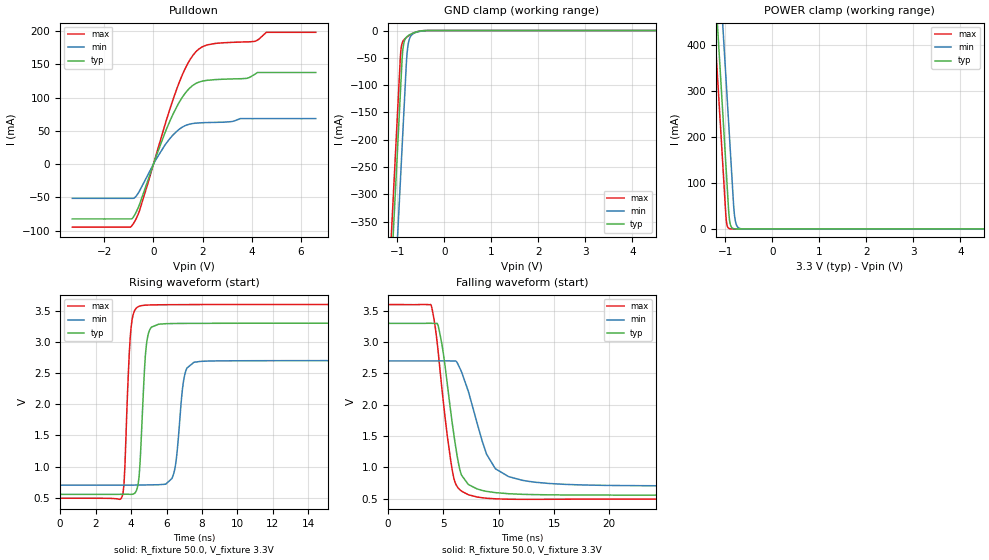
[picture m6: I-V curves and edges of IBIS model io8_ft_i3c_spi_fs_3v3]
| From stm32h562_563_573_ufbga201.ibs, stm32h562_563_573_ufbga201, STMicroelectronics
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[Model]   io8_ft_i3c_spi_fs_3v3
Model_type I/O_open_drain
Polarity   Non-Inverting
Enable   Active-Low
| CAP_THRESHOLD on pad IOFT is "UDTCAPC" :
| Rising=20.0% of vddiom   Falling=80.0% of vddiom
| C_comp min and max val. don't necessarily correlate with the min and max pvt
| but are the smallest and greatest pad capacitance found.
| var   typ   min   max
C_comp   3.95818pF  3.95027pF  4.00766pF
|C_comp_pulldown   3.95818pF  3.95027pF  4.00766pF
Vinl = 1.35V
Vinh = 1.8V
Vmeas = 1.65V   | Reference voltage for timing measurements
Cref  = 50.0pF   | Timing specification test load capacitance value
Rref  = 1.0MOhm   | Timing specification test load resistance value
Vref  = 1.815V   | Timing specification test load voltage
[Model Spec]
| TIME_THRESHOLD on pin ZII2CV11 is "CMOS" :
| Rising=40.0% of vdd   Falling=60.0% of vdd
Vinl 1.29880V 1.07480V 1.40680V
Vinh 1.77520V 1.49320V 1.89720V
| variable   typ   min   max
[Temperature Range] 25.0 125.0 -40.0
| variable   typ   min   max
[Voltage Range] 3.3V 2.7V 3.6V
| variable   typ   min   max
[POWER Clamp Reference] 3.3V 2.7V 3.6V
| variable   typ   min   max
[GND Clamp Reference] 0V 0V 0V
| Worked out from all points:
|   slope of the pulldown table from 0 to 0.495 V, typ, clamps not added: 10 ohm
|   GND clamp passes 1 mA (typ) near -0.52 V on its own axis
|   POWER clamp passes 1 mA (typ) near -0.84 V on its own axis
|   rising waveform, R_fixture 50.0, V_fixture 3.3V: 20-80 % time 285ps typ, 381ps min, 266ps max; typ from 0.556 V to 3.3 V
|   falling waveform, R_fixture 50.0, V_fixture 3.3V: 20-80 % time 1.27ns typ, 2.18ns min, 1.21ns max; typ from 3.3 V to 0.556 V
[POWER Clamp]
-3.3V     4.068A     4.259A     3.957A
-1.25V    582.8mA    774.2mA    471.5mA
-1.21V    514.8mA    706.2mA    403.5mA
-1.13V    378.8mA    570.2mA    267.5mA
-1.04V    225.8mA    417.2mA    114.5mA
-980mV    123.8mA    315.2mA    17.95mA
-920mV    26.3mA     213.2mA    906uA
-880mV    5.543mA    145.2mA    123.7uA
-810mV    363.5uA    33.6mA     3.798uA
-770mV    76.62uA    10.47mA    519.4nA
-690mV    3.409uA    1.017mA    10.46nA
6.6V      0A         0A         0A
[GND Clamp]
-3.3V     -4.13A     -4.291A    -4.063A
-1.25V    -644.7mA   -806.4mA   -578.1mA
-940mV    -117.7mA   -279.4mA   -51.06mA
-920mV    -83.75mA   -245.4mA   -31.43mA
-900mV    -50.5mA    -211.4mA   -23.14mA
-880mV    -31.27mA   -177.4mA   -19.1mA
-850mV    -18.68mA   -126.4mA   -15.73mA
-800mV    -11.46mA   -46.4mA    -12.03mA
-760mV    -8.752mA   -20.02mA   -9.606mA
-680mV    -5.122mA   -6.673mA   -5.579mA
-300mV    -5.379uA   -47.63uA   -852.7nA
6.6V      10.49nA    1.843uA    393.6pA
| variable   typ   min   max
[Pullup Reference] 3.3V 2.7V 3.6V
| variable   typ   min   max
[Pulldown Reference] 0V 0V 0V
[Pulldown]
-3.3V     -82.42mA   -51.49mA   -94.82mA
-850mV    -81.27mA   -51.49mA   -91.26mA
-580mV    -62.01mA   -41.36mA   -71.41mA
120mV     12.61mA    7.999mA    15.37mA
800mV     75.3mA     43.94mA    97.52mA
1.33V     108.3mA    58.37mA    146.5mA
1.84V     123.1mA    61.83mA    172.7mA
2.51V     126.9mA    62.7mA     181.3mA
3.78V     128.8mA    68.32mA    183.7mA
4.12V     134.9mA    68.32mA    184.6mA
4.59V     137.6mA    68.32mA    198mA
6.6V      137.6mA    68.32mA    198mA
[Ramp]
dV/dt_r 1.64659V/283.08007ps 1.1979V/378.52865ps 1.86382V/262.83024ps
dV/dt_f 1.64666V/1.26939ns 1.19801V/2.06853ns 1.86387V/1.20927ns
R_load = 50.0
| Removed startup time: 0s 0s 0s  .
| Removed end time: 19.4ns.
[Rising Waveform]
R_fixture   = 50.0
V_fixture   = 3.3V
V_fixture_min = 2.7V
V_fixture_max = 3.6V
0s        555.6mV    703.3mV    493.6mV
3.5ns     556.9mV    703.5mV    526.5mV
3.95ns    556.1mV    704mV      3.066V
4.4ns     724.9mV    705.1mV    3.565V
4.8ns     2.76V      706.8mV    3.589V
5.15ns    3.237V     708.6mV    3.593V
6.35ns    3.295V     842.7mV    3.597V
7ns       3.297V     2.44V      3.598V
7.55ns    3.297V     2.674V     3.599V
19.4ns    3.3V       2.7V       3.6V
| Removed startup time: 0s 0s 0s  .
| Removed end time: 59.35ns.
[Falling Waveform]
R_fixture   = 50.0
V_fixture   = 3.3V
V_fixture_min = 2.7V
V_fixture_max = 3.6V
0s        3.3V       2.7V       3.6V
3.9ns     3.301V     2.7V       3.587V
4.7ns     3.121V     2.7V       2.546V
5.85ns    1.643V     2.699V     906.3mV
6.5ns     954.5mV    2.579V     639.7mV
7.3ns     721.3mV    2.187V     559.7mV
8.9ns     616.1mV    1.21V      506.4mV
9.7ns     595.4mV    976.7mV    496.8mV
12.6ns    566.4mV    778.4mV    488.6mV
59.35ns   555.6mV    703.3mV    493.6mV
